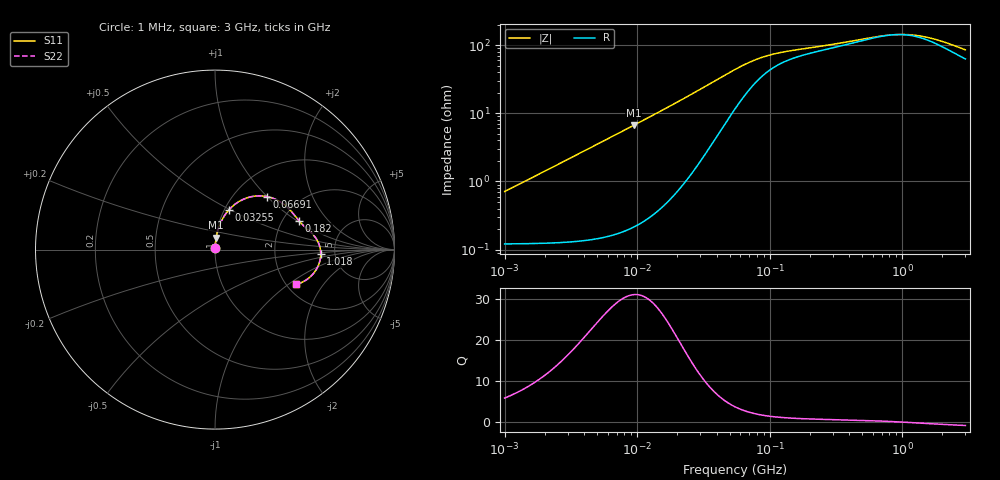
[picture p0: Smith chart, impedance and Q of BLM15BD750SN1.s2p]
! BLM15BD750SN1
# Hz S RI R 50
!Freq.(Hz) S11(Real) S11(Imag) S21(Real) S21(Imag) S12(Real) S12(Imag) S22(Real) S22(Imag)
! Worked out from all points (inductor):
!   401 points, 1 MHz to 3 GHz, reference 50 ohm
!   read as one part in series: L = 111 nH near 1.041 MHz
!   highest Q = 31.1 at 9.41 MHz (marker M1), where L = 112 nH
!   self-resonance near 879.2 MHz
!   S11 on the Smith chart (normalised r, x): 1 MHz: 1.00, +0.01; 32.55 MHz: 1.05, +0.49; 66.91 MHz: 1.40, +0.99; 182 MHz: 2.44, +1.04; 1.018 GHz: 3.85, -0.30; 3 GHz: 2.25, -1.15
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1000000  0.00126 0.00698  0.9987 -0.00698  0.9987 -0.00698  0.00126 0.00698
1246295  0.00129 0.0087  0.9987 -0.0087  0.9987 -0.0087  0.00129 0.0087
3823119  0.00205 0.0267  0.9979 -0.0267  0.9979 -0.0267  0.00205 0.0267
9410094  0.00649 0.0659  0.9935 -0.0659  0.9935 -0.0659  0.00649 0.0659
1.461624e7  0.0144 0.1024  0.9856 -0.1024  0.9856 -0.1024  0.0144 0.1024
2.316168e7  0.0369 0.1616  0.9631 -0.1616  0.9631 -0.1616  0.0369 0.1616
3.254976e7  0.0772 0.221  0.9228 -0.221  0.9228 -0.221  0.0772 0.221
4.22235e7  0.134 0.2679  0.866 -0.2679  0.866 -0.2679  0.134 0.2679
5.477226e7  0.2168 0.2973  0.7832 -0.2973  0.7832 -0.2973  0.2168 0.2973
6.690963e7  0.2879 0.2958  0.7121 -0.2958  0.7121 -0.2958  0.2879 0.2958
8.338914e7  0.3558 0.2708  0.6442 -0.2708  0.6442 -0.2708  0.3558 0.2708
1.018679e8  0.4003 0.2383  0.5997 -0.2383  0.5997 -0.2383  0.4003 0.2383
1.295243e8  0.4351 0.2009  0.5649 -0.2009  0.5649 -0.2009  0.4351 0.2009
1.820241e8  0.467 0.1609  0.533 -0.1609  0.533 -0.1609  0.467 0.1609
2.094008e8  0.4782 0.1482  0.5218 -0.1482  0.5218 -0.1482  0.4782 0.1482
4.75755e8  0.5472 0.0828  0.4528 -0.0828  0.4528 -0.0828  0.5472 0.0828
8.005644e8  0.5841 0.0155  0.4159 -0.0155  0.4159 -0.0155  0.5841 0.0155
1.017911e9  0.5892 -0.0258  0.4108 0.0258  0.4108 0.0258  0.5892 -0.0258
1.294266e9  0.5823 -0.0707  0.4177 0.0707  0.4177 0.0707  0.5823 -0.0707
1.67892e9  0.5593 -0.119  0.4407 0.119  0.4407 0.119  0.5593 -0.119
2.312676e9  0.5086 -0.1687  0.4914 0.1687  0.4914 0.1687  0.5086 -0.1687
3e9  0.4538 -0.1937  0.5462 0.1937  0.5462 0.1937  0.4538 -0.1937
